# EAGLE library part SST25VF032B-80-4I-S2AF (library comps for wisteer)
SST25VF032B-50-4I-S2AF: Flash memory (32Mbits) http://ww1.microchip.com/downloads/en/DeviceDoc/25071A.pdf
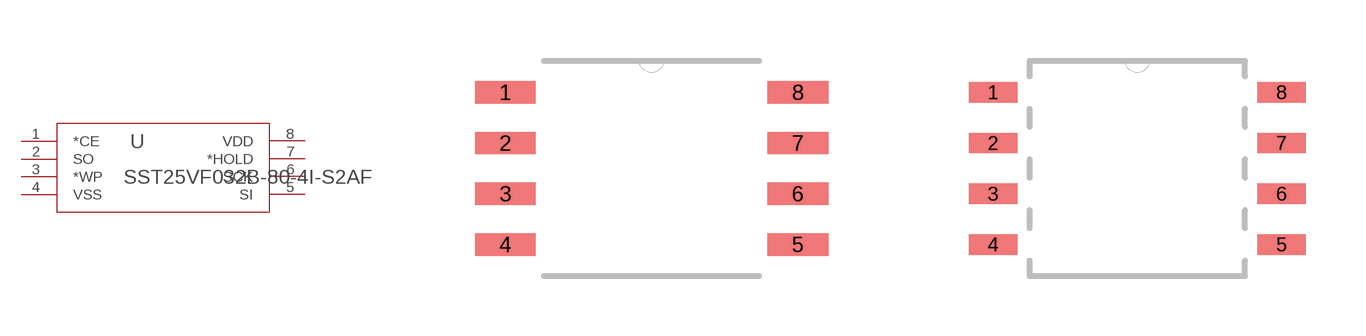
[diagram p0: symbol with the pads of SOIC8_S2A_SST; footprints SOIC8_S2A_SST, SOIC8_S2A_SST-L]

Designator prefix -

## SST25VF032B-80-4I-S2AF (MANUFACTURER_PART_NUMBER: sst25vf032b-80-4i-s2af; VENDOR: Microchip)  [SOIC8_S2A_SST]
1  *CE  in
2  SO  out
3  *WP  in
4  VSS  pwr
5  SI  in
6  SCK  in
7  *HOLD  in
8  VDD  pwr

## SST25VF032B-80-4I-S2AFL  [SOIC8_S2A_SST-L]
Pads as for SOIC8_S2A_SST

## SST25VF032B-80-4I-S2AFM  [SOIC8_S2A_SST-M]
Pads as for SOIC8_S2A_SST

## Footprint SOIC8_S2A_SST (pad centres in mm)
smd 1.524 x 0.559: 1 -3.658,1.905; 2 -3.658,0.635; 3 -3.658,-0.635; 4 -3.658,-1.905; 5 3.658,-1.905; 6 3.658,-0.635; 7 3.658,0.635; 8 3.658,1.905

## Footprint SOIC8_S2A_SST-L (pad centres in mm)
smd 1.219 x 0.508: 1 -3.607,1.905; 2 -3.607,0.635; 3 -3.607,-0.635; 4 -3.607,-1.905; 5 3.607,-1.905; 6 3.607,-0.635; 7 3.607,0.635; 8 3.607,1.905

## Footprint SOIC8_S2A_SST-M (pad centres in mm)
smd 1.829 x 0.61: 1 -3.708,1.905; 2 -3.708,0.635; 3 -3.708,-0.635; 4 -3.708,-1.905; 5 3.708,-1.905; 6 3.708,-0.635; 7 3.708,0.635; 8 3.708,1.905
